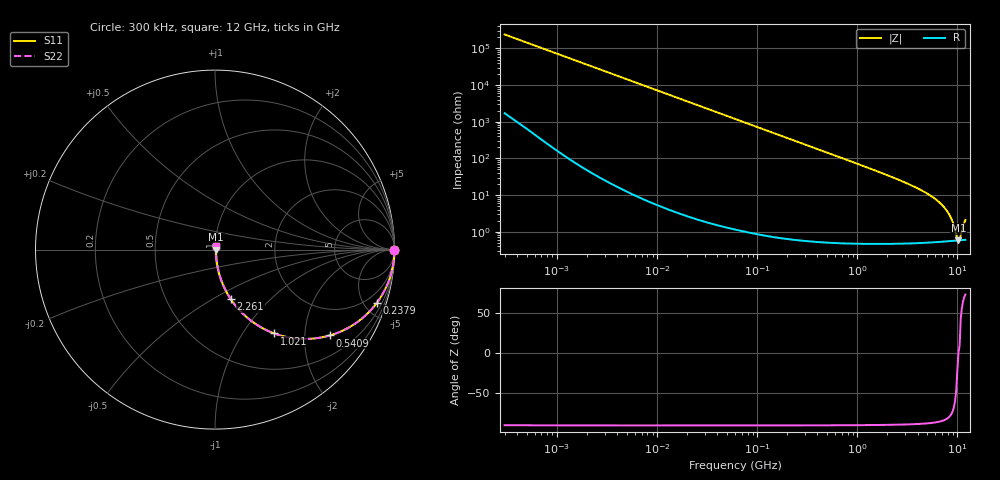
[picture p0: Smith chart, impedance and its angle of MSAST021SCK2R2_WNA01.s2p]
! MSAST021SCK2R2_WNA01  S-PARAMETER MODEL  ( General Type )
! Model Generated by TAIYO YUDEN Corporation (http://www.ty-top.com)
! Version 2.0
! TAIYO YUDEN Control No. 181101
! Copyright(c) 2015 TAIYO YUDEN CO.,LTD. All Rights Reserved.
! Product Description (link to TY-COMPAS)
! https://ds.yuden.co.jp/TYCOMPAS/or/detail?pn=MSAST021SCK2R2BWNA01&u=M
! Products Name : Multilayer Ceramic Capacitors
! Characteristics :
!  Capacitance : 2.2 pF , Rated Voltage : 25V , TCC : CK / C0K
!  Case Size : 0.25 x 0.125 / 0.0098 x 0.0049 [mm/inch] , Thickness : 0.125 / 0.0049 [mm/inch]
!  (Conditions: Temperature = 25 degC , DC Bias Current/Voltage = 0A / 0V)
! External Node Assignments :
!  1  o---| |---o  2
! GND o---------o GND
! Frequency Range : 0.3MHz  -  12000MHz  [ 401 STEP ]
# MHz S RI R 50
! Freq[MHz].  S11 Real  S11 Imag  S21 Real  S21 Imag  S12 Real  S12 Imag  S22 Real  S22 Imag
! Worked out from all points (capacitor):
!   401 points, 300 kHz to 12 GHz, reference 50 ohm
!   read as one part in series: C = 2.2 pF near 316.3 kHz
!   lowest |Z| = 580 mohm at 10.24 GHz (marker M1)
!   series resonance near 10.23 GHz, so ESL is about 110 pH
!   S11 on the Smith chart (normalised r, x): 300 kHz: open; 237.9 MHz: 1.01, -6.08; 540.9 MHz: 1.01, -2.67; 1.021 GHz: 1.01, -1.40; 2.261 GHz: 1.01, -0.61; 12 GHz: 1.01, +0.04
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0.3  1 -0.000415  3.12e-06 0.000415  3.12e-06 0.000415  1 -0.000415
1.769972  1 -0.00245  9.46e-06 0.00245  9.46e-06 0.00245  1 -0.00245
10.44266  0.9998 -0.0144  0.000219 0.0144  0.000219 0.0144  0.9998 -0.0144
60  0.9931 -0.0824  0.00691 0.0824  0.00691 0.0824  0.9931 -0.0824
122.6847  0.9718 -0.1648  0.0282 0.1648  0.0282 0.1648  0.9718 -0.1648
237.9135  0.9018 -0.2966  0.0982 0.2966  0.0982 0.2966  0.9018 -0.2966
353.9943  0.8058 -0.3943  0.1942 0.3943  0.1942 0.3943  0.8058 -0.3943
540.8523  0.6397 -0.4782  0.3603 0.4782  0.3603 0.4782  0.6397 -0.4782
743.2595  0.4839 -0.4973  0.5161 0.4973  0.5161 0.4973  0.4839 -0.4973
1021.415  0.3306 -0.4671  0.6694 0.4671  0.6694 0.4671  0.3306 -0.4671
2088.533  0.1025 -0.2963  0.8975 0.2963  0.8975 0.2963  0.1025 -0.2963
2261.293  0.0881 -0.2759  0.9119 0.2759  0.9119 0.2759  0.0881 -0.2759
4385.161  0.0223 -0.1304  0.9777 0.1304  0.9777 0.1304  0.0223 -0.1304
6699.894  0.00888 -0.0599  0.9911 0.0599  0.9911 0.0599  0.00888 -0.0599
7448.838  0.00733 -0.044  0.9927 0.044  0.9927 0.044  0.00733 -0.044
8281.503  0.00632 -0.0286  0.9937 0.0286  0.9937 0.0286  0.00632 -0.0286
8966.534  0.0059 -0.0173  0.9941 0.0173  0.9941 0.0173  0.0059 -0.0173
9968.853  0.00574 -0.00223  0.9943 0.00223  0.9943 0.00223  0.00574 -0.00223
10236.47  0.00577 6.32e-05  0.9942 -6.32e-05  0.9942 -6.32e-05  0.00577 6.32e-05
10793.46  0.00588 0.00568  0.9941 -0.00568  0.9941 -0.00568  0.00588 0.00568
11380.75  0.00607 0.0125  0.9939 -0.0125  0.9939 -0.0125  0.00607 0.0125
12000  0.00637 0.0197  0.9936 -0.0197  0.9936 -0.0197  0.00637 0.0197
